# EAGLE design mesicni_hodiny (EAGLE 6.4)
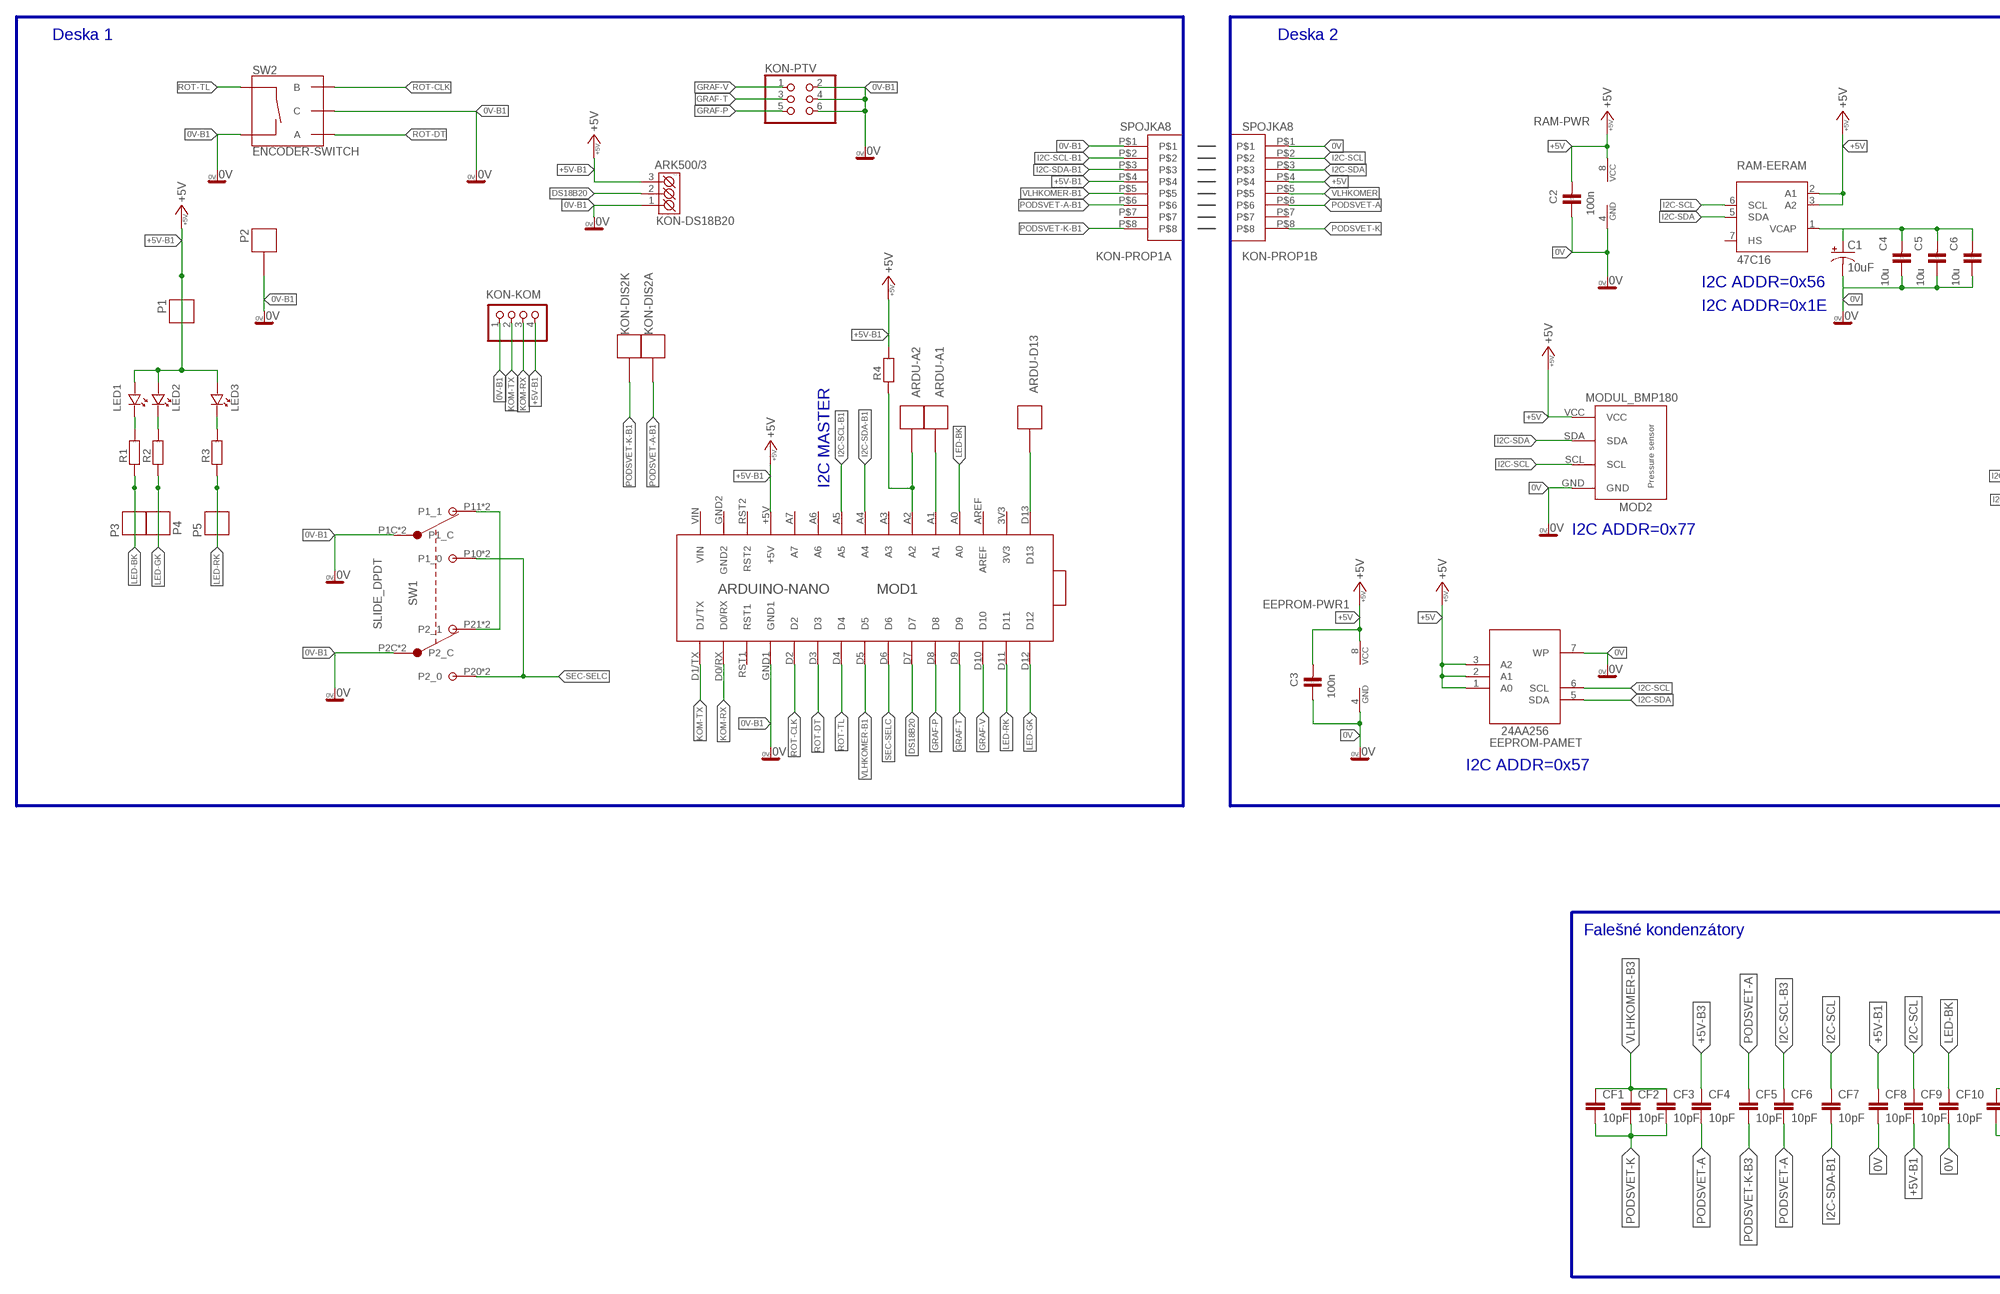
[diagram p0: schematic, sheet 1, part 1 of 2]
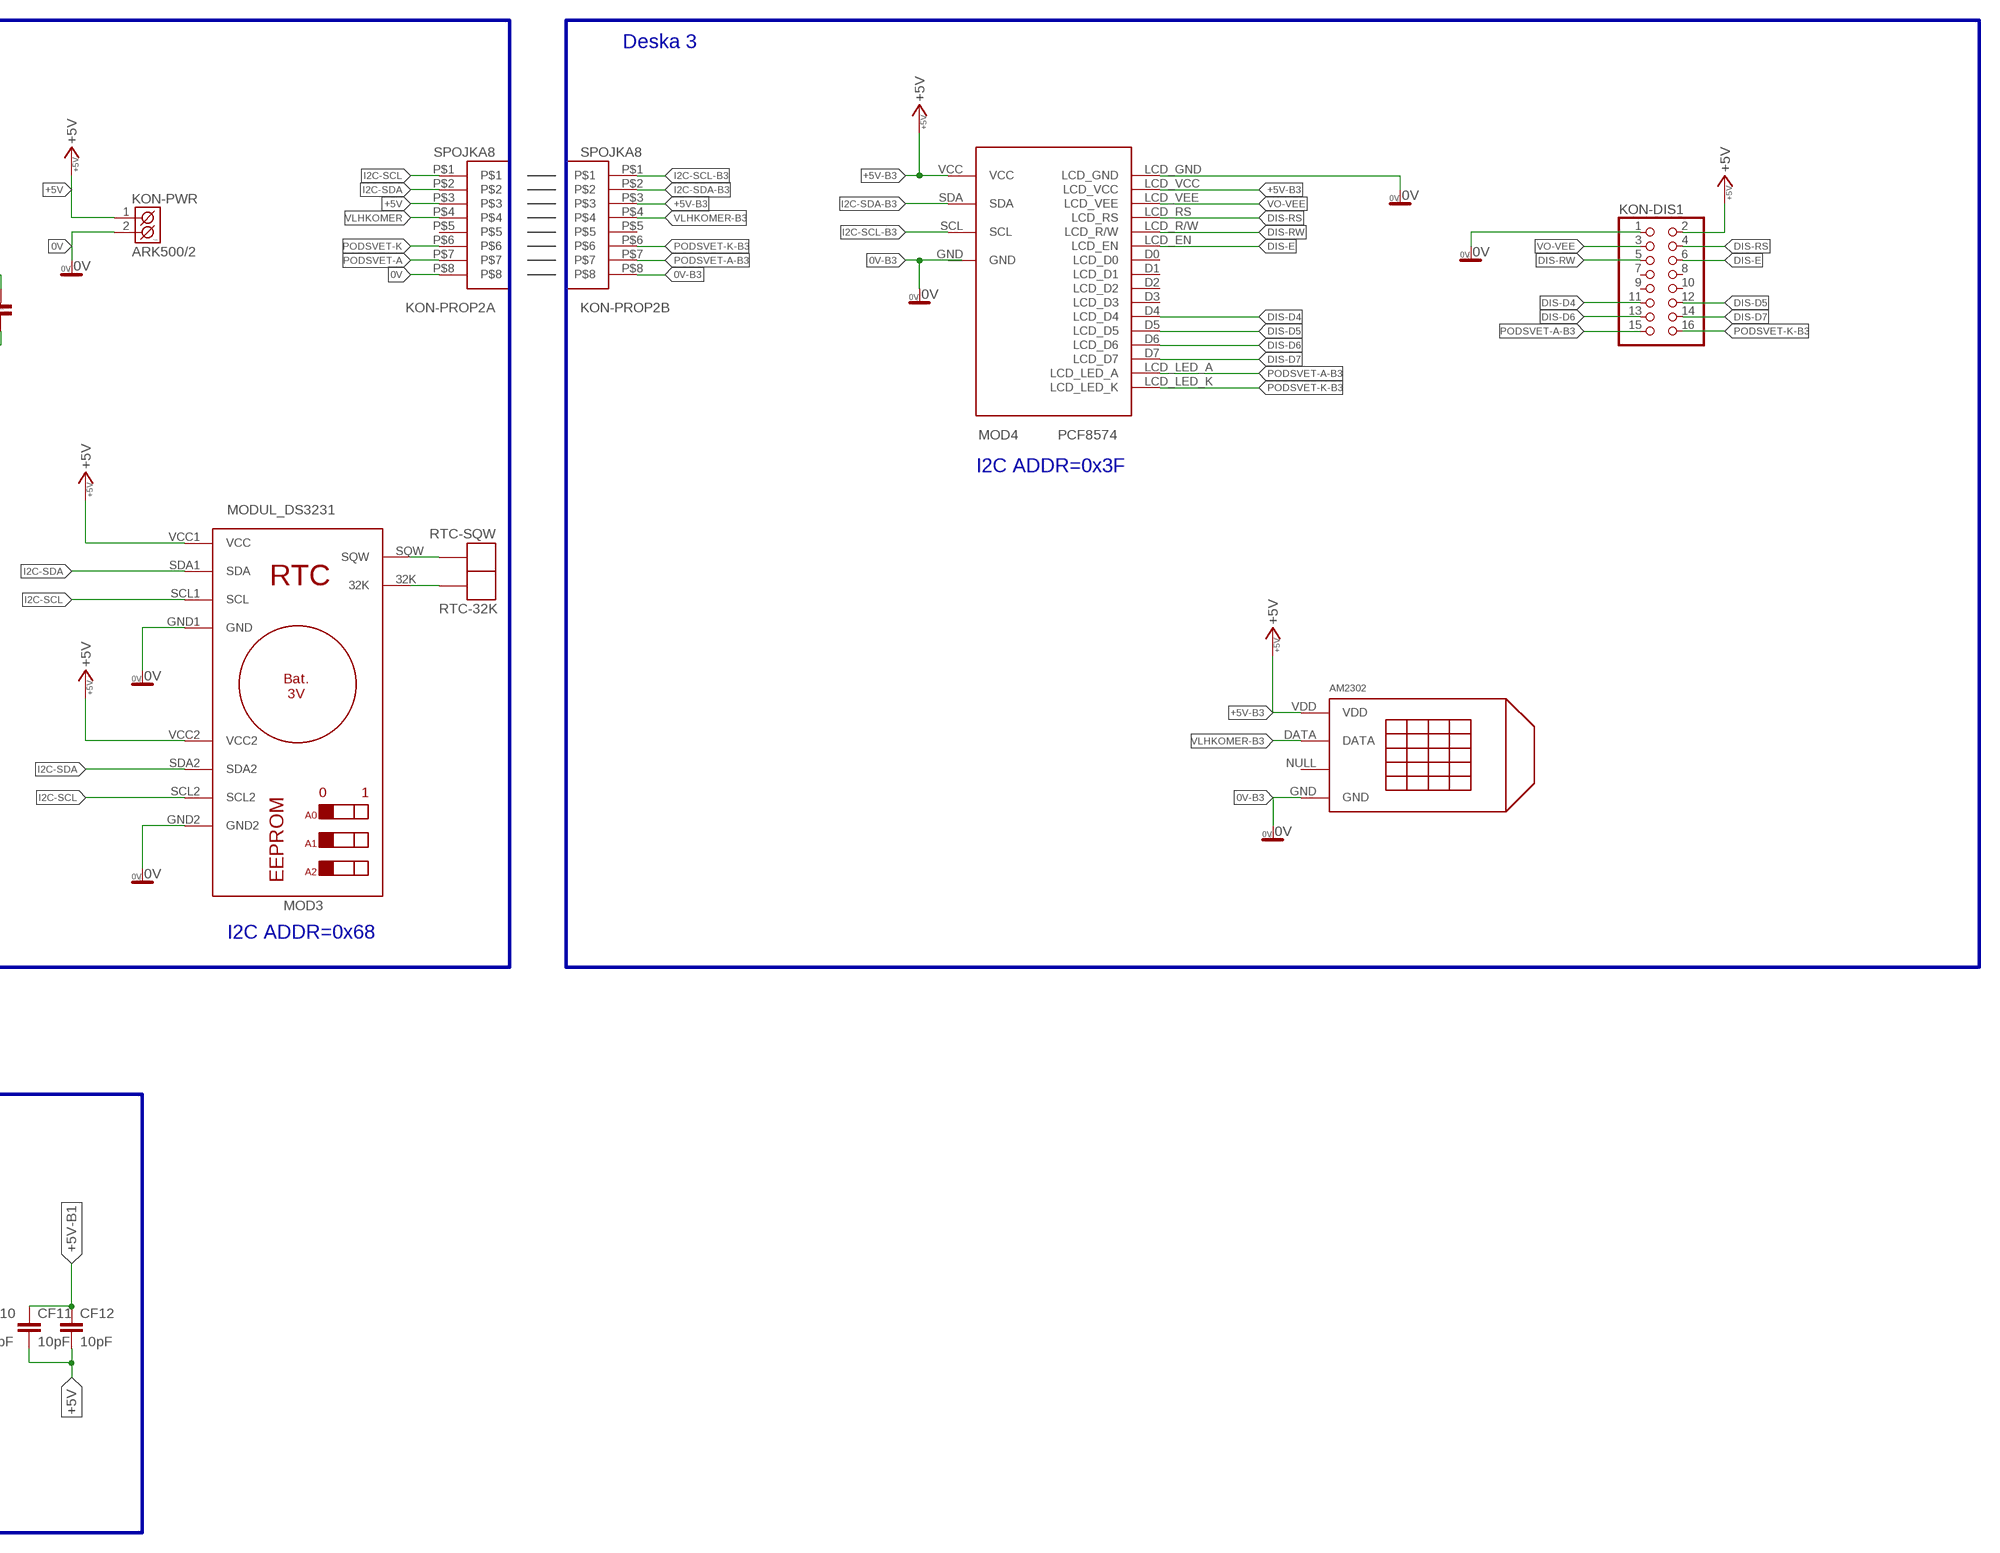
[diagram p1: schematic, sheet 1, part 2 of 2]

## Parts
AM2302  RHT03_DHT-22_AM2302RA  [RHT03_DHT-22/RA]
ARDU-A1  BIGPIN  [BIGPIN]
ARDU-A2  BIGPIN  [BIGPIN]
ARDU-D13  BIGPIN  [BIGPIN]
C1  10uF  10UF-POLAR-RADIAL-2.5MM-25V-20%  [CPOL-RADIAL-2.5MM-5MM]
C2  100n  C-KERAMIK_SMD_0805  [0805]
C3  100n  C-KERAMIK_SMD_0805  [0805]
C4  10u  C-KERAMIK_SMD_0805  [0805]
C5  10u  C-KERAMIK_SMD_0805  [0805]
C6  10u  C-KERAMIK_SMD_0805  [0805]
CF1  10pF  10PF-0603-50V-5%  [0603]
CF2  10pF  10PF-0603-50V-5%  [0603]
CF3  10pF  10PF-0603-50V-5%  [0603]
CF4  10pF  10PF-0603-50V-5%  [0603]
CF5  10pF  10PF-0603-50V-5%  [0603]
CF6  10pF  10PF-0603-50V-5%  [0603]
CF7  10pF  10PF-0603-50V-5%  [0603]
CF8  10pF  10PF-0603-50V-5%  [0603]
CF9  10pF  10PF-0603-50V-5%  [0603]
CF10  10pF  10PF-0603-50V-5%  [0603]
CF11  10pF  10PF-0603-50V-5%  [0603]
CF12  10pF  10PF-0603-50V-5%  [0603]
EEPROM  24AA256  EEPROMP  [DIL08]
KON-DIS1  PINHD-2X8  [2X08]
KON-DIS2A  BIGPIN  [BIGPIN]
KON-DIS2K  BIGPIN  [BIGPIN]
KON-DS18B20  ARK500/3  [ARK500/3]
KON-KOM  PINHD-1X4  [1X04]
KON-PROP1A  SPOJKA8  [SPOJKA8]
KON-PROP1B  SPOJKA8  [SPOJKA8]
KON-PROP2A  SPOJKA8  [SPOJKA8]
KON-PROP2B  SPOJKA8  [SPOJKA8]
KON-PTV  PINHD-2X3  [2X03]
KON-PWR  ARK500/2  [ARK500/2]
LED1  LED_3  [LED_3]
LED2  LED_3  [LED_3]
LED3  LED_3  [LED_3]
MOD1  ARDUINO-NANO  [PDIP-32]
MOD2  MODUL_BMP180  [MODUL_BMP180]
MOD3  MODUL_DS3231  [DS3231]
MOD4  PCF8574  I2C_DISPLAY_BACKPACK  [I2C_DISPLAY_BACKPACK]
P1  BIGPIN  [BIGPIN]
P2  BIGPIN  [BIGPIN]
P3  BIGPIN  [BIGPIN]
P4  BIGPIN  [BIGPIN]
P5  BIGPIN  [BIGPIN]
R1  R_SMD_0805  [0805]
R2  R_SMD_0805  [0805]
R3  R_SMD_0805  [0805]
R4  R_SMD_0805  [0805]
RAM  47C16  PCA8581CT  [SO08]
RTC-32K  BIGPIN  [BIGPIN]
RTC-SQW  BIGPIN  [BIGPIN]
SW1  SLIDE_DPDT  [SLIDE_DPDT]
SW2  ENCODER-SWITCH  [ROTARY_ENC_PLAIN]

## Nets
0V: C1.2(-) C2.1 C3.1 C4.1 C5.1 C6.1 CF8.2 CF10.2 EEPROM.4(-PWR1:GND) EEPROM.7(-PAMET:WP) KON-PROP1B.P$1 KON-PROP2A.P$8 KON-PWR.2(K2) MOD2.GND MOD3.GND1(GND) MOD3.GND2 RAM.4(-PWR:GND)
0V-B1: KON-DS18B20.1(K1) KON-KOM.1 KON-PROP1A.P$1 KON-PTV.2 KON-PTV.4 KON-PTV.6 MOD1.GND1 P2.P$1 SW1.P1C(P1_C) SW1.P1CSMD(P1_C) SW1.P2C(P2_C) SW1.P2CSMD(P2_C) SW2.C SW2.SW- ; supply symbol labelled 0V
0V-B3: AM2302.GND KON-DIS1.1 KON-PROP2B.P$8 MOD4.GND MOD4.LCD_GND ; supply symbol labelled 0V
+5V: C2.2 C3.2 CF11.2 CF12.2 EEPROM.1(-PAMET:A0) EEPROM.2(-PAMET:A1) EEPROM.3(-PAMET:A2) EEPROM.8(-PWR1:VCC) KON-PROP1B.P$4 KON-PROP2A.P$3 KON-PWR.1(K1) MOD2.VCC MOD3.VCC1(VCC) MOD3.VCC2 RAM.2(-EERAM:A1) RAM.3(-EERAM:A2) RAM.8(-PWR:VCC)
+5V-B1: CF8.1 CF9.2 CF11.1 CF12.1 KON-DS18B20.3(K3) KON-KOM.4 KON-PROP1A.P$4 LED1.A LED2.A LED3.A MOD1.+5V P1.P$1 R4.2 ; supply symbol labelled +5V
+5V-B3: AM2302.VDD CF4.1 KON-DIS1.2 KON-PROP2B.P$3 MOD4.LCD_VCC MOD4.VCC ; supply symbol labelled +5V
A1: ARDU-A1.P$1 MOD1.A1
DIS-D4: KON-DIS1.11 MOD4.D4(LCD_D4)
DIS-D5: KON-DIS1.12 MOD4.D5(LCD_D5)
DIS-D6: KON-DIS1.13 MOD4.D6(LCD_D6)
DIS-D7: KON-DIS1.14 MOD4.D7(LCD_D7)
DIS-E: KON-DIS1.6 MOD4.LCD_EN
DIS-RS: KON-DIS1.4 MOD4.LCD_RS
DIS-RW: KON-DIS1.5 MOD4.LCD_R/W
DS18B20: KON-DS18B20.2(K2) MOD1.D7
GRAF-P: KON-PTV.5 MOD1.D8
GRAF-T: KON-PTV.3 MOD1.D9
GRAF-V: KON-PTV.1 MOD1.D10
I2C-SCL: CF7.1 CF9.1 EEPROM.6(-PAMET:SCL) KON-PROP1B.P$2 KON-PROP2A.P$1 MOD2.SCL MOD3.SCL1(SCL) MOD3.SCL2 RAM.6(-EERAM:SCL)
I2C-SCL-B1: KON-PROP1A.P$2 MOD1.A5
I2C-SCL-B3: CF6.1 KON-PROP2B.P$1 MOD4.SCL
I2C-SDA: EEPROM.5(-PAMET:SDA) KON-PROP1B.P$3 KON-PROP2A.P$2 MOD2.SDA MOD3.SDA1(SDA) MOD3.SDA2 RAM.5(-EERAM:SDA)
I2C-SDA-B1: CF7.2 KON-PROP1A.P$3 MOD1.A4
I2C-SDA-B3: KON-PROP2B.P$2 MOD4.SDA
KOM-RX: KON-KOM.3 MOD1.D0/RX
KOM-TX: KON-KOM.2 MOD1.D1/TX
LED-BK: CF10.1 MOD1.A0 P3.P$1 R1.1
LED-GK: MOD1.D12 P4.P$1 R2.1
LED-RK: MOD1.D11 P5.P$1 R3.1
N$1: LED1.K R1.2
N$2: LED2.K R2.2
N$3: LED3.K R3.2
N$5: MOD3.SQW RTC-SQW.P$1
N$7: MOD3.32K RTC-32K.P$1
N$8: ARDU-D13.P$1 MOD1.D13
N$9: ARDU-A2.P$1 MOD1.A2 R4.1
N$17: C1.1(+) C4.2 C5.2 C6.2 RAM.1(-EERAM:VCAP)
NIC-1: SW1.P11(P1_1) SW1.P11SMD(P1_1) SW1.P21(P2_1) SW1.P21SMD(P2_1)
PODSVET-A: CF4.2 CF5.1 CF6.2 KON-PROP1B.P$6 KON-PROP2A.P$7
PODSVET-A-B1: KON-DIS2A.P$1 KON-PROP1A.P$6
PODSVET-A-B3: KON-DIS1.15 KON-PROP2B.P$7 MOD4.LCD_LED_A
PODSVET-K: CF1.2 CF2.2 CF3.2 KON-PROP1B.P$8 KON-PROP2A.P$6
PODSVET-K-B1: KON-DIS2K.P$1 KON-PROP1A.P$8
PODSVET-K-B3: CF5.2 KON-DIS1.16 KON-PROP2B.P$6 MOD4.LCD_LED_K
ROT-CLK: MOD1.D2 SW2.B
ROT-DT: MOD1.D3 SW2.A
ROT-TL: MOD1.D4 SW2.SW+
SEC-SELC: MOD1.D6 SW1.P10(P1_0) SW1.P10SMD(P1_0) SW1.P20(P2_0) SW1.P20SMD(P2_0)
VLHKOMER: KON-PROP1B.P$5 KON-PROP2A.P$4
VLHKOMER-B1: KON-PROP1A.P$5 MOD1.D5
VLHKOMER-B3: AM2302.DATA CF1.1 CF2.1 CF3.1 KON-PROP2B.P$4
VO-VEE: KON-DIS1.3 MOD4.LCD_VEE
Unconnected: AM2302.NULL KON-DIS1.7 KON-DIS1.8 KON-DIS1.9 KON-DIS1.10 KON-PROP1A.P$7 KON-PROP1B.P$7 KON-PROP2A.P$5 KON-PROP2B.P$5 MOD1.3V3 MOD1.A3 MOD1.A6 MOD1.A7 MOD1.AREF MOD1.GND2 MOD1.RST1 MOD1.RST2 MOD1.VIN MOD4.D0(LCD_D0) MOD4.D1(LCD_D1) MOD4.D2(LCD_D2) MOD4.D3(LCD_D3) RAM.7(-EERAM:HS)

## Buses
B$1
B$2
B$3
B$4

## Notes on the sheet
- Deska 1 | Deska 2 | Deska 3
- I2C ADDR=0x56
- I2C ADDR=0x1E
- I2C ADDR=0x3F
- I2C MASTER
- I2C ADDR=0x77
- I2C ADDR=0x57
- I2C ADDR=0x68
- Falešné kondenzátory

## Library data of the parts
AM2302 = RHT03_DHT-22_AM2302:RHT03_DHT-22_AM2302: RHT03 / DHT-22 / AM2302 Packages and symbol for the RHT03 / DHT-22 relative humidity and temperature sensor. Note: The AM2302 is a wired version of the DHT-22 which typically requires less clearance and is thus provided as a separate package.; PROD_ID: SEN-10167
ARDU-A1 ARDU-A2 ARDU-D13 KON-DIS2A KON-DIS2K P1-P5 RTC-32K RTC-SQW = bigpin:BIGPIN: Jeden ovalny pin
C1 = SparkFun-Capacitors:10UF-POLAR: 10.0µF polarized capacitors; PROD_ID: CAP-08440
C2-C6 = #PaJa_30:C-KERAMIK: Kondenzator - keramicky
CF1-CF12 = SparkFun-Capacitors:10PF: 10pF ceramic capacitors; PROD_ID: CAP-11812
EEPROM = eeprom:EEPROM: EEPROM
KON-DIS1 = pinhead:PINHD-2X8: PIN HEADER
KON-DS18B20 = #PaJa_konektory:ARK500/3: Svorkovnice - roztec 5mm - trojita
KON-KOM = pinhead:PINHD-1X4: PIN HEADER
KON-PROP1A KON-PROP1B KON-PROP2A KON-PROP2B = spopjka8:SPOJKA8
KON-PTV = pinhead:PINHD-2X3: PIN HEADER
KON-PWR = #PaJa_konektory:ARK500/2: Svorkovnice - roztec 5mm - dvojita
LED1-LED3 = #PaJa_30:LED: LED - jednobarevna
MOD1 = jet-lib:ARDUINO-NANO: Arduino NANO - V3
MOD2 = modul_bmp180:MODUL_BMP180
MOD3 = modul_DS3231:MODUL_DS3231: Modul DS3231 s externi pameti
MOD4 = i2c_display_backpack:I2C_DISPLAY_BACKPACK
R1-R4 = #PaJa_30:R: Rezistor
RAM = i2c:PCA8581: 2048 x 8-Bit EERAM with I²C Bus Interface
SW1 = slide_DPDT:SLIDE_DPDT
SW2 = SparkFun-Switches:ENCODER-SWITCH: Rotary Encoder w/ Select Switch Encoders rotate similarly to potentiometers, but they’re different from potentiometers in that an encoder has full rotation without limits. They output gray code so that you can tell how much and in which direction the encoder has been turned. This encoder includes a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; SF_SKU: COM-09117

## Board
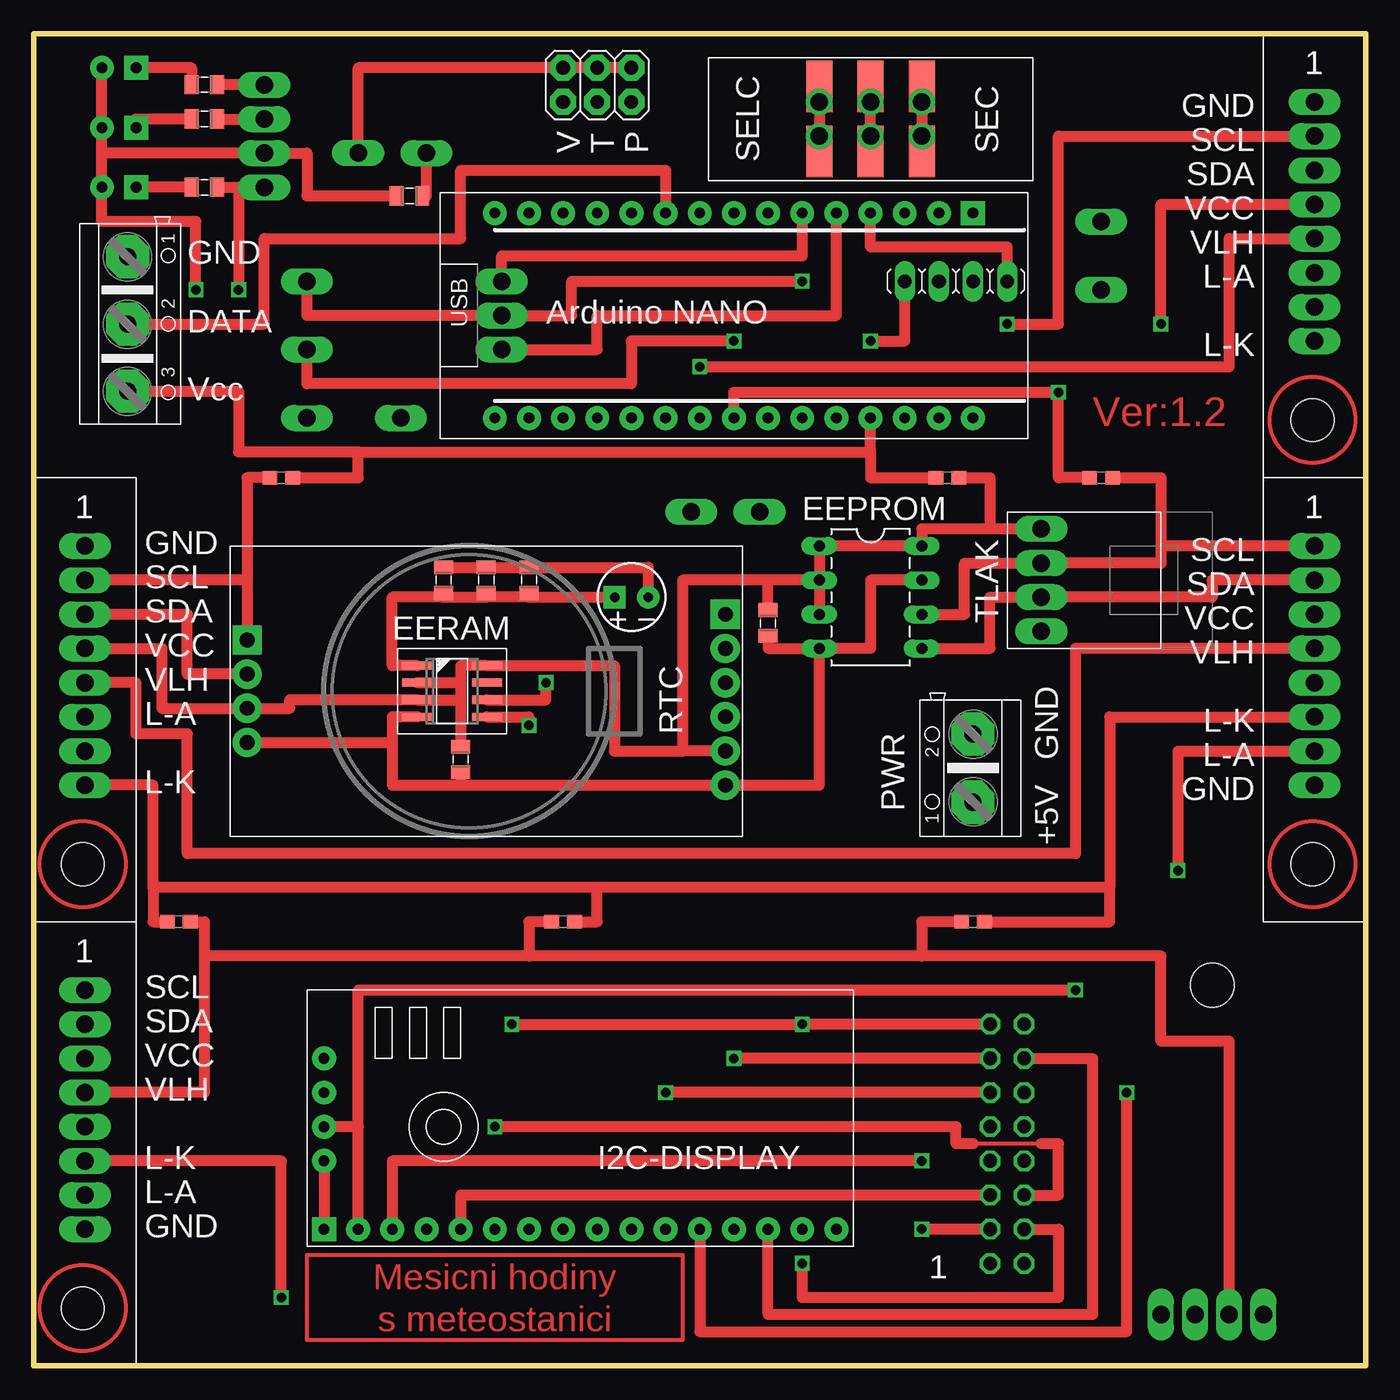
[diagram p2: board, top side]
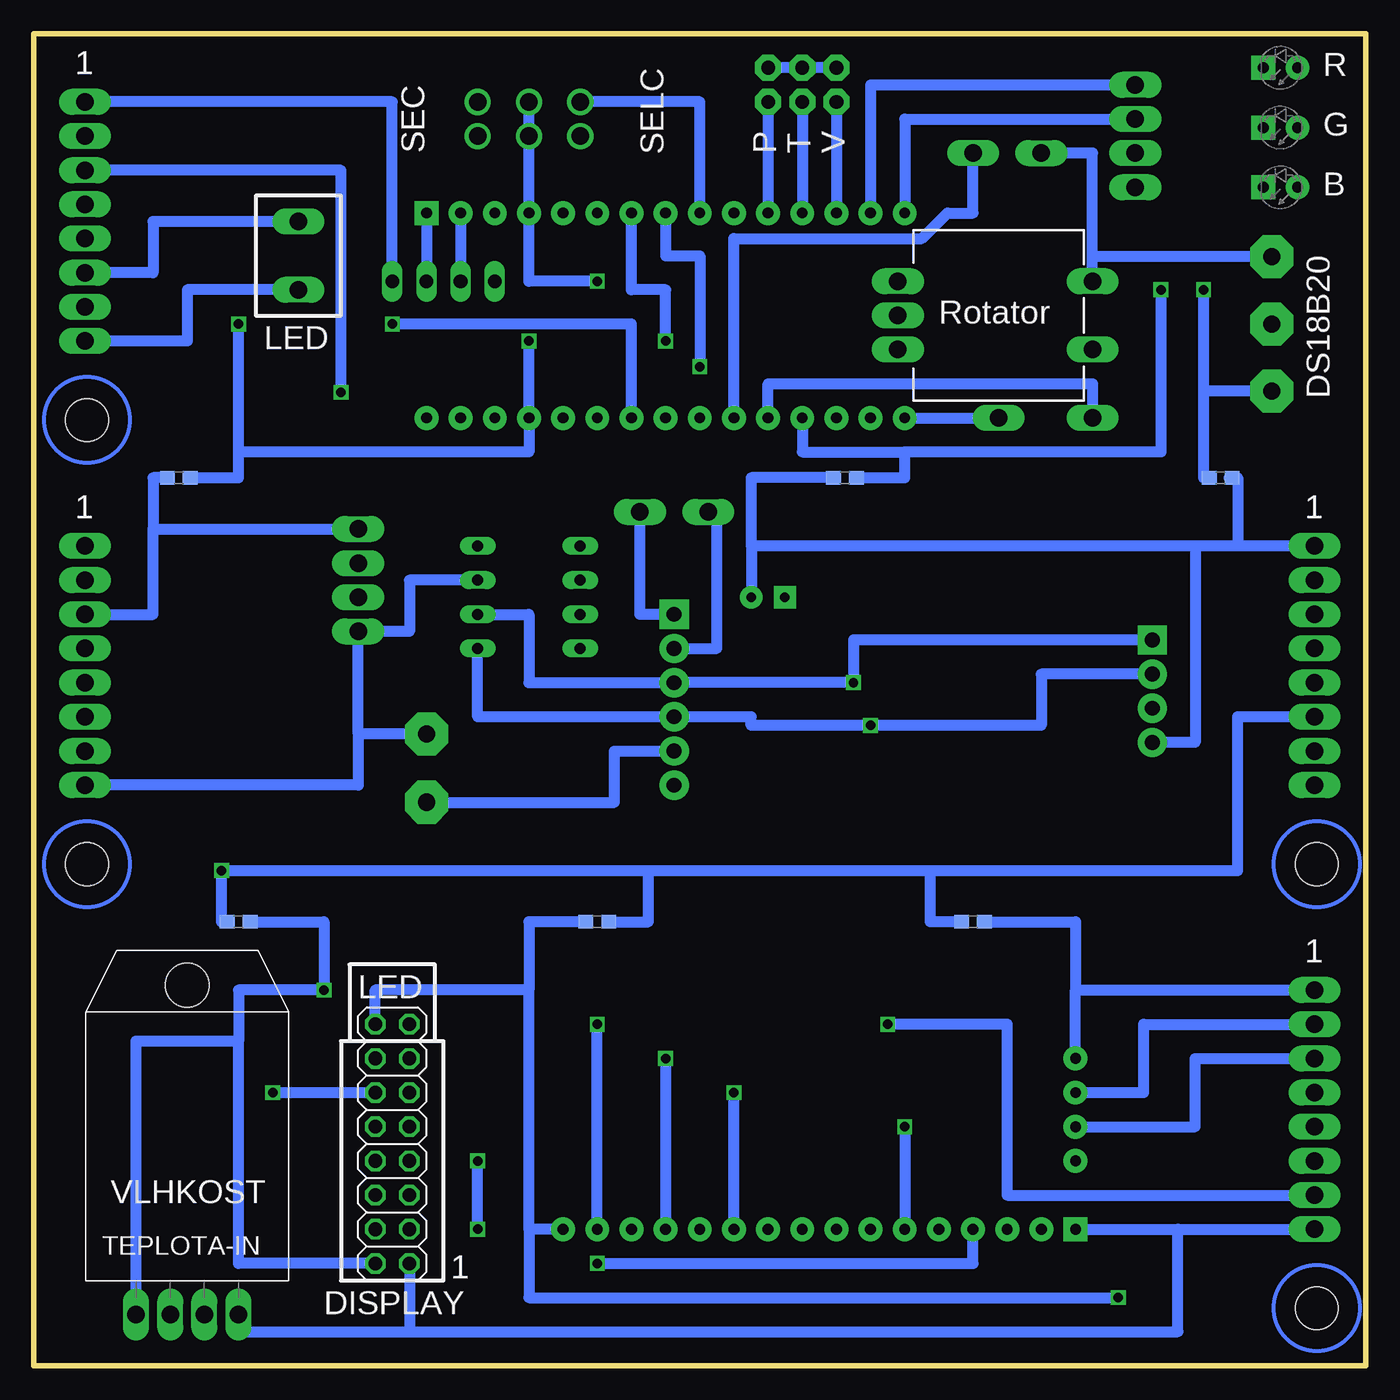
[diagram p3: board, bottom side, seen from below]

Size 99.06 x 99.06 mm. Coordinates in mm from the lower left corner, seen from the top.
Outline: 0,99.06 99.06,99.06 99.06,0 0,0 0,99.06
Copper layers (1*16): Top 0.035mm / dielectric 1.5mm / Bottom 0.035mm
Design rules "default *": minimum track width 10mil, minimum drill 24mil, track to track 8mil, track to pad 8mil, pad to pad 8mil, via to via 8mil, smd to smd 8mil, copper to edge 40mil, drill to drill 8mil, minimum pad ring 10mil, minimum via ring 8mil, stop-mask expansion 4mil, vias tented up to drill 0mil, thermal gap 10mil

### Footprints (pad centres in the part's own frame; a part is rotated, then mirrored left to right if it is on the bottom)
RHT03_DHT-22/RA = drill 1.3 pad 1.778 long: DATA -1.27,0; GND 3.81,0; NULL 1.27,0; VDD -3.81,0 | hole 3.25: 0,24.5
BIGPIN = drill 1.3 long: P$1 0,0
CPOL-RADIAL-2.5MM-5MM = drill 0.7 pad 1.651 square: 1 1.25,0 | drill 0.7 pad 1.651: 2 -1.25,0
0805 = smd 1.016 x 1.422: 1 -0.953,0; 2 0.953,0
0603 = smd 1.1 x 1: 1 -0.85,0; 2 0.85,0
DIL08 = drill 0.813 long: 1 -3.81,-3.81; 2 -1.27,-3.81; 3 1.27,-3.81; 4 3.81,-3.81; 5 3.81,3.81; 6 1.27,3.81; 7 -1.27,3.81; 8 -3.81,3.81
2X08 = drill 1.016 octagon: 1 -8.89,-1.27; 2 -8.89,1.27; 3 -6.35,-1.27; 4 -6.35,1.27; 5 -3.81,-1.27; 6 -3.81,1.27; 7 -1.27,-1.27; 8 -1.27,1.27; 9 1.27,-1.27; 10 1.27,1.27; 11 3.81,-1.27; 12 3.81,1.27; 13 6.35,-1.27; 14 6.35,1.27; 15 8.89,-1.27; 16 8.89,1.27
ARK500/3 = drill 1.27 pad 3.2 octagon: 1 -5,0; 2 0,0; 3 5,0
1X04 = drill 1.016 long: 1 -3.81,0; 2 -1.27,0; 3 1.27,0; 4 3.81,0
SPOJKA8 = drill 1.3 pad 1.778 long: P$1 0,8.89; P$2 0,6.35; P$3 0,3.81; P$4 0,1.27; P$5 0,-1.27; P$6 0,-3.81; P$7 0,-6.35; P$8 0,-8.89 | hole 3.2: -0.159,-14.764
2X03 = drill 1.016 pad 1.93 octagon: 1 -2.54,-1.27; 2 -2.54,1.27; 3 0,-1.27; 4 0,1.27; 5 2.54,-1.27; 6 2.54,1.27
ARK500/2 = drill 1.27 pad 3.2 octagon: 1 -2.54,0; 2 2.54,0
LED_3 = drill 0.813 pad 1.778: A -1.27,0 | drill 0.813 pad 1.778 square: K 1.27,0
PDIP-32 = drill 0.8 pad 1.778: 3V3 15.24,-35.56; +5V 15.24,-10.16; A0 15.24,-30.48; A1 15.24,-27.94; A2 15.24,-25.4; A3 15.24,-22.86; A4 15.24,-20.32; A5 15.24,-17.78; A6 15.24,-15.24; A7 15.24,-12.7; AREF 15.24,-33.02; D0/RX 0,-5.08; D2 0,-12.7; D3 0,-15.24; D4 0,-17.78; D5 0,-20.32; D6 0,-22.86; D7 0,-25.4; D8 0,-27.94; D9 0,-30.48; D10 0,-33.02; D11 0,-35.56; D12 0,-38.1; D13 15.24,-38.1; GND1 0,-10.16; GND2 15.24,-5.08; RST1 0,-7.62; RST2 15.24,-7.62; VIN 15.24,-2.54 | drill 0.8 pad 1.778 square: D1/TX 0,-2.54
MODUL_BMP180 = drill 1.3 pad 1.778 long: GND -3.81,3.81; SCL 1.27,3.81; SDA -1.27,3.81; VCC 3.81,3.81
DS3231 = drill 1.1 pad 2.184 square: 32K 36.83,16.51; SCL1 1.27,14.605 | drill 1.1 pad 2.184: GND1 1.27,6.985; GND2 36.83,3.81; SCL2 36.83,11.43; SDA1 1.27,12.065; SDA2 36.83,8.89; SQW 36.83,13.97; VCC1 1.27,9.525; VCC2 36.83,6.35
I2C_DISPLAY_BACKPACK = drill 0.8 pad 1.778: D0 5.08,7.62; D1 2.54,7.62; D2 0,7.62; D3 -2.54,7.62; D4 -5.08,7.62; D5 -7.62,7.62; D6 -10.16,7.62; D7 -12.7,7.62; GND 20.32,2.54; LCD_EN 7.62,7.62; LCD_LED_A -15.24,7.62; LCD_LED_K -17.78,7.62; LCD_R/W 10.16,7.62; LCD_RS 12.7,7.62; LCD_VCC 17.78,7.62; LCD_VEE 15.24,7.62; SCL 20.32,-5.08; SDA 20.32,-2.54; VCC 20.32,0 | drill 0.8 pad 1.778 square: LCD_GND 20.32,7.62
SO08 = smd 0.6 x 2.2: 1 -1.905,-2.6; 2 -0.635,-2.6; 3 0.635,-2.6; 4 1.905,-2.6; 5 1.905,2.6; 6 0.635,2.6; 7 -0.635,2.6; 8 -1.905,2.6
SLIDE_DPDT = drill 1.3: P1C -1.27,0; P2C 1.27,0; P10 -1.27,3.81; P11 -1.27,-3.81; P20 1.27,3.81; P21 1.27,-3.81 | smd 3.81 x 1.93: P1CSMD -2.413,0; P2CSMD 2.413,0; P10SMD -2.413,3.81; P11SMD -2.413,-3.81; P20SMD 2.413,3.81; P21SMD 2.413,-3.81
ROTARY_ENC_PLAIN = drill 1.3 pad 1.778 long: A 7.493,-2.54; B 7.493,2.54; C 7.493,0; SW+ -6.985,2.54; SW- -6.985,-2.54

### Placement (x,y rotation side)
AM2302  87.63,3.81 0 bottom
ARDU-A1  20.32,70.48 0 top
ARDU-A2  29.21,90.17 0 top
ARDU-D13  27.3,70.48 0 top
C1  44.45,57.15 180 top
C2  31.75,45.09 90 top
C3  54.61,55.24 90 top
C4  36.83,58.42 270 top
C5  33.66,58.42 270 top
C6  30.48,58.42 270 top
CF1  10.79,33.02 180 top
CF2  39.37,33.02 0 top
CF3  69.85,33.02 0 top
CF4  83.82,33.02 180 bottom
CF5  57.15,33.02 180 bottom
CF6  29.21,33.02 180 bottom
CF7  79.38,66.04 180 top
CF8  10.79,66.04 0 bottom
CF9  18.41,66.04 0 top
CF10  38.73,66.04 180 bottom
CF11  67.94,66.04 0 top
CF12  88.27,66.04 180 bottom
EEPROM  62.23,57.15 270 top
KON-DIS1  72.39,16.51 90 bottom
KON-DIS2A  79.38,85.09 0 top
KON-DIS2K  79.38,80.01 0 top
KON-DS18B20  6.99,77.47 270 top
KON-KOM  68.58,80.64 180 top
KON-PROP1A  95.25,85.09 0 top
KON-PROP1B  3.81,52.07 0 top
KON-PROP2A  95.25,52.07 0 top
KON-PROP2B  3.81,19.05 0 top
KON-PTV  41.91,95.25 0 top
KON-PWR  69.85,44.45 90 top
LED1  6.35,87.63 180 bottom
LED2  6.35,92.08 180 bottom
LED3  6.35,96.52 180 bottom
MOD1  72.39,85.72 270 top
MOD2  78.74,58.42 90 top
MOD3  14.61,39.37 0 top
MOD4  41.91,17.78 180 top
P1  17.14,90.17 0 top
P2  24.13,90.17 180 top
P3  17.14,87.63 0 top
P4  17.14,92.71 0 top
P5  17.14,95.25 0 top
R1  12.7,87.63 180 top
R2  12.7,92.71 180 top
R3  12.7,95.25 180 top
R4  27.94,87 180 top
RAM  31.11,50.16 270 top
RTC-32K  53.98,63.5 180 top
RTC-SQW  48.9,63.5 180 top
SW1  62.23,92.71 90 top
SW2  27.3,78.11 180 bottom

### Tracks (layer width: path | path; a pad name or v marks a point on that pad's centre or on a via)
0V
  Top 0.813: EEPROM.7 62.23,58.42 62.23,53.34 EEPROM.4 | EEPROM.4 58.42,43.18 MOD3.GND2 31.75,43.18 | RAM.4 26.67,48.26 26.67,46.35 | 26.67,46.35 26.67,43.18 31.75,43.18 | MOD3.GND1 26.67,46.35 | C2.1 31.75,43.18 | C3.1 54.61,53.34 EEPROM.4 | C6.1 C5.1 C4.1 45.7,59.37 C1.2
  Bottom 0.813: 74.93,46.99 MOD2.GND 71.12,54.61 71.12,58.42 EEPROM.7 | 12.7,60.96 12.7,46.35 MOD3.GND1 | KON-PROP2A.P$8 74.93,43.18 74.93,46.99 | KON-PROP1B.P$1 9.53,60.96 | 10.16,66.04 CF8.2 9.53,66.04 9.53,60.96 | 9.53,60.96 12.7,60.96 | CF10.2 45.7,66.04 45.7,60.96 | KON-PWR.2 74.93,46.99 | 12.7,60.96 45.7,60.96 | 45.7,60.96 C1.2
0V-B1  (via drill 0.7)
  Top 0.813: v57.15,80.64 40.01,80.64 40.01,78.11 SW2.C 20.32,78.11 SW2.SW- | P2.P$1 24.13,96.52 KON-PTV.6 | SW1.P1CSMD SW1.P1C SW1.P2C SW1.P2CSMD | KON-KOM.1 72.39,83.19 62.23,83.19 MOD1.GND1
  Bottom 0.813: v57.15,80.64 62.23,80.64 MOD1.GND1 SW1.P2C | KON-KOM.1 72.39,93.98 KON-PROP1A.P$1 | KON-PTV.2 KON-PTV.4 KON-PTV.6 | 20.32,82.47 20.32,90.17 P2.P$1 | KON-DS18B20.1 20.32,82.47 | SW2.SW- 20.32,82.47
0V-B3
  Top 0.813: MOD4.GND MOD4.LCD_GND
  Bottom 0.813: AM2302.GND 83.82,2.54 71.12,2.54 | 71.12,2.54 13.97,2.54 13.97,10.16 | MOD4.LCD_GND 13.97,10.16 | 13.97,10.16 KON-PROP2B.P$8 | KON-DIS1.1 71.12,2.54
+5V
  Top 0.813: MOD2.VCC 71.12,62.23 | 71.12,62.23 66.04,62.23 EEPROM.8 EEPROM.1 EEPROM.2 | EEPROM.2 EEPROM.3 | EEPROM.2 54.61,58.42 | 54.61,58.42 48.26,58.42 48.26,45.72 | 48.26,45.72 43.18,45.72 43.18,52.07 RAM.8 31.75,52.07 31.75,50.8 | MOD3.VCC2 48.26,45.72 | KON-PROP1B.P$4 9.53,53.34 9.53,48.9 MOD3.VCC1 19.05,48.9 19.05,49.53 RAM.3 31.75,49.53 | 31.75,50.8 31.75,49.53 | 31.75,49.53 C2.2 | C3.2 54.61,58.42 | RAM.2 31.75,50.8 | CF11.2 71.12,66.04 71.12,62.23
  Bottom 0.813: KON-PROP2A.P$3 90.17,55.88 90.17,62.23 | 90.17,62.23 MOD2.VCC | CF12.2 90.17,66.04 90.17,62.23 | KON-PWR.1 55.88,41.91 55.88,45.72 MOD3.VCC2
+5V-B1  (via drill 0.7)
  Top 0.813: v83.82,77.47 83.82,86.36 KON-PROP1A.P$4 | KON-DS18B20.3 15.24,72.47 15.24,67.94 24.13,67.94 | 24.13,67.94 62.23,67.94 | 62.23,67.94 MOD1.+5V | v12.06,80.01 12.06,85.09 5.08,85.09 LED1.A 5.08,90.17 | CF9.2 24.13,66.04 24.13,67.94 | 62.23,67.94 62.23,66.04 CF11.1 | v62.23,76.2 64.77,76.2 KON-KOM.4 | 5.08,90.17 LED2.A LED3.A | 5.08,90.17 P1.P$1 20.32,90.17 20.32,87 R4.2
  Bottom 0.813: 83.82,67.94 62.23,67.94 MOD1.+5V v62.23,76.2 | 83.82,67.94 v83.82,77.47 | KON-DS18B20.3 12.06,72.47 | 12.06,72.47 v12.06,80.01 | CF8.1 12.06,66.04 12.06,72.47 | CF12.1 83.82,66.04 83.82,67.94
+5V-B3  (via drill 0.7)
  Top 0.813: 24.13,17.78 MOD4.VCC | 24.13,17.78 24.13,27.94 v77.47,27.94 | MOD4.LCD_VCC 24.13,17.78
  Bottom 0.813: MOD4.VCC 12.7,17.78 12.7,22.86 KON-PROP2B.P$3 | 83.82,24.13 83.82,27.94 v77.47,27.94 77.47,33.02 CF4.1 | 83.82,24.13 91.44,24.13 AM2302.VDD | 83.82,24.13 83.82,7.62 KON-DIS1.2
A1
  Bottom 0.813: MOD1.A1 44.45,73.03 20.32,73.03 ARDU-A1.P$1
DIS-D4  (via drill 0.7)
  Top 0.813: KON-DIS1.11 v46.99,20.32
  Bottom 0.813: MOD4.D4 v46.99,20.32
DIS-D5  (via drill 0.7)
  Top 0.813: MOD4.D5 49.53,2.54 81.28,2.54 v81.28,20.32
  Bottom 0.813: v81.28,20.32 KON-DIS1.12
DIS-D6  (via drill 0.7)
  Top 0.813: KON-DIS1.13 v52.07,22.86
  Bottom 0.813: v52.07,22.86 MOD4.D6
DIS-D7
  Top 0.813: KON-DIS1.14 78.74,22.86 78.74,3.81 54.61,3.81 MOD4.D7
DIS-E  (via drill 0.7)
  Top 0.305: 74.93,16.51 69.85,16.51
  Top 0.813: KON-DIS1.6 76.2,12.7 76.2,16.51 74.93,16.51 | 69.85,16.51 68.58,16.51 68.58,17.78 v34.29,17.78
  Bottom 0.813: v34.29,17.78 MOD4.LCD_EN
DIS-RS  (via drill 0.7)
  Top 0.813: KON-DIS1.4 76.2,10.16 76.2,5.08 57.15,5.08 v57.15,7.62
  Bottom 0.813: v57.15,7.62 29.21,7.62 MOD4.LCD_RS
DIS-RW
  Top 0.813: KON-DIS1.5 31.75,12.7 MOD4.LCD_R/W
DS18B20
  Top 0.813: KON-DS18B20.2 17.14,77.47 17.14,83.82 31.75,83.82 31.75,88.9 46.99,88.9 MOD1.D7
GRAF-P
  Bottom 0.813: KON-PTV.5 MOD1.D8
GRAF-T
  Bottom 0.813: KON-PTV.3 MOD1.D9
GRAF-V
  Bottom 0.813: KON-PTV.1 MOD1.D10
I2C-SCL  (via drill 0.7)
  Top 0.813: KON-PROP2A.P$1 83.82,60.96 | 83.82,60.96 83.82,59.69 MOD2.SCL 69.22,59.69 69.22,55.88 EEPROM.6 | v38.1,50.8 38.1,49.53 RAM.6 | 15.88,58.42 MOD3.SCL1 | 15.88,58.42 KON-PROP1B.P$2 | CF9.1 15.88,66.04 15.88,58.42 | CF7.1 83.82,66.04 83.82,60.96
  Bottom 0.813: EEPROM.6 62.23,55.88 62.23,50.8 MOD3.SCL2 v38.1,50.8 38.1,53.98 MOD3.SCL1
I2C-SCL-B1  (via drill 0.7)
  Top 0.813: v72.39,77.47 76.2,77.47 76.2,91.44 KON-PROP1A.P$2
  Bottom 0.813: MOD1.A5 54.61,77.47 v72.39,77.47
I2C-SCL-B3
  Bottom 0.813: MOD4.SCL 21.59,27.94 | 21.59,27.94 KON-PROP2B.P$1 | CF6.1 21.59,33.02 21.59,27.94
I2C-SDA  (via drill 0.7)
  Top 0.813: KON-PROP2A.P$2 87.63,58.42 87.63,57.15 MOD2.SDA 71.12,57.15 71.12,53.34 EEPROM.5 | MOD3.SDA1 11.43,51.44 11.43,55.88 KON-PROP1B.P$3 | v36.83,47.62 36.83,48.26 RAM.5
  Bottom 0.813: MOD3.SDA1 24.13,51.44 24.13,47.62 v36.83,47.62 45.72,47.62 45.72,48.26 MOD3.SDA2 66.04,48.26 EEPROM.5
I2C-SDA-B1  (via drill 0.7)
  Top 0.813: MOD1.A4 52.07,72.39 v76.2,72.39 76.2,66.04 CF7.2
  Bottom 0.813: v76.2,72.39 76.2,88.9 KON-PROP1A.P$3
I2C-SDA-B3
  Bottom 0.813: MOD4.SDA 16.51,20.32 16.51,25.4 KON-PROP2B.P$2
KOM-RX
  Bottom 0.813: MOD1.D0/RX KON-KOM.3
KOM-TX
  Bottom 0.813: MOD1.D1/TX KON-KOM.2
LED-BK  (via drill 0.7)
  Top 0.813: R1.1 P3.P$1 15.24,87.63 v15.24,80.01
  Bottom 0.813: v15.24,80.01 15.24,67.94 34.29,67.94 | CF10.1 34.29,66.04 34.29,67.94 | MOD1.A0 41.91,67.94 34.29,67.94
LED-GK
  Top 0.813: R2.1 P4.P$1
  Bottom 0.813: MOD1.D12 34.29,92.71 P4.P$1
LED-RK
  Top 0.813: P5.P$1 R3.1
  Bottom 0.813: MOD1.D11 36.83,95.25 P5.P$1
N$1
  Top 0.813: R1.2 LED1.K
N$2
  Top 0.813: R2.2 7.62,92.71 LED2.K
N$3
  Top 0.813: R3.2 11.75,96.52 LED3.K
N$4
  Top 0.305: 20.32,8.26 48.26,8.26 48.26,1.91 20.32,1.91 20.32,8.26
N$5
  Bottom 0.813: MOD3.SQW 48.26,53.34 48.26,63.5 RTC-SQW.P$1
N$7
  Bottom 0.813: MOD3.32K 53.98,55.88 RTC-32K.P$1
N$8
  Bottom 0.813: MOD1.D13 ARDU-D13.P$1
N$9
  Top 0.813: R4.1 29.21,87 ARDU-A2.P$1
  Bottom 0.813: MOD1.A2 46.99,83.82 33.02,83.82 31.11,85.72 29.21,85.72 ARDU-A2.P$1
N$17
  Top 0.813: 36.83,57.15 C1.1 | RAM.1 26.67,52.07 26.67,57.15 30.48,57.15 | C4.2 36.83,57.15 | 36.83,57.15 33.66,57.15 | C6.2 30.48,57.15 | 30.48,57.15 33.66,57.15 | 33.66,57.15 C5.2
NIC-1
  Top 0.813: SW1.P11SMD SW1.P11 SW1.P21 SW1.P21SMD
PODSVET-A  (via drill 0.7)
  Top 0.813: v85.09,36.83 85.09,45.72 KON-PROP2A.P$7
  Bottom 0.813: 53.34,36.83 v85.09,36.83 85.09,33.02 CF4.2 | 53.34,36.83 32.38,36.83 | 32.38,36.83 9.53,36.83 9.53,48.26 KON-PROP1B.P$6 | CF5.1 53.34,33.02 53.34,36.83 | CF6.2 32.38,33.02 32.38,36.83
PODSVET-A-B1
  Bottom 0.813: KON-DIS2A.P$1 90.17,85.09 90.17,81.28 KON-PROP1A.P$6
PODSVET-A-B3  (via drill 0.7)
  Top 0.813: v35.56,25.4 v57.15,25.4 KON-DIS1.15
  Bottom 0.813: v35.56,25.4 26.67,25.4 26.67,12.7 KON-PROP2B.P$7 | MOD4.LCD_LED_A v57.15,25.4
PODSVET-K
  Top 0.813: 80.01,35.56 80.01,48.26 KON-PROP2A.P$6 | 80.01,35.56 41.91,35.56 | 41.91,35.56 8.89,35.56 | 8.89,35.56 8.89,43.18 KON-PROP1B.P$8 | 8.89,35.56 8.89,33.02 CF1.2 | CF2.2 41.91,33.02 41.91,35.56 | CF3.2 80.01,33.02 80.01,35.56
PODSVET-K-B1
  Bottom 0.813: KON-PROP1A.P$8 87.63,76.2 87.63,80.01 KON-DIS2K.P$1
PODSVET-K-B3  (via drill 0.7)
  Top 0.813: v18.41,5.08 18.41,15.24 KON-PROP2B.P$6
  Bottom 0.813: 62.23,10.16 62.23,27.94 | 62.23,27.94 73.66,27.94 KON-DIS1.16 | MOD4.LCD_LED_K 62.23,10.16 | 62.23,10.16 62.23,5.08 v18.41,5.08 | CF5.2 62.23,33.02 62.23,27.94
ROT-CLK
  Top 0.813: SW2.B 41.91,75.56 41.91,78.11 59.69,78.11 MOD1.D2
ROT-DT
  Top 0.813: MOD1.D3 57.15,82.55 34.8,82.55 SW2.A
ROT-TL  (via drill 0.7)
  Top 0.813: v52.07,76.2 44.45,76.2 44.45,73.03 20.32,73.03 SW2.SW+
  Bottom 0.813: v52.07,76.2 52.07,80.01 54.61,80.01 MOD1.D4
SEC-SELC
  Top 0.813: SW1.P20SMD SW1.P20 SW1.P10 SW1.P10SMD
  Bottom 0.813: MOD1.D6 49.53,93.98 SW1.P20
VLHKOMER
  Top 0.813: KON-PROP2A.P$4 77.47,53.34 77.47,38.1 11.43,38.1 11.43,46.99 7.62,46.99 7.62,50.8 KON-PROP1B.P$5
VLHKOMER-B1  (via drill 0.7)
  Top 0.813: v49.53,74.3 88.9,74.3 88.9,83.82 KON-PROP1A.P$5
  Bottom 0.813: MOD1.D5 52.07,82.55 49.53,82.55 v49.53,74.3
VLHKOMER-B3
  Top 0.813: AM2302.DATA 88.9,24.13 83.82,24.13 83.82,30.48 66.04,30.48 | 66.04,30.48 36.83,30.48 | 36.83,30.48 12.7,30.48 | 12.7,30.48 12.7,20.32 KON-PROP2B.P$4 | CF1.1 12.7,33.02 12.7,30.48 | CF2.1 36.83,33.02 36.83,30.48 | CF3.1 66.04,33.02 66.04,30.48
VO-VEE  (via drill 0.7)
  Top 0.813: KON-DIS1.3 v66.04,10.16 | v66.04,15.24 26.67,15.24 MOD4.LCD_VEE
  Bottom 0.813: v66.04,10.16 v66.04,15.24

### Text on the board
Top: Ver:1.2 | Mesicni hodiny / s meteostanici
tPlace: 1 | GND | SCL | V | T | P | SELC | SEC | SDA | VCC | VLH | GND | L-A | DATA | Arduino NANO | L-K | Vcc | 1 | 1 | EEPROM | SCL | GND | SDA | SCL | VCC | SDA | TLAK | EERAM | VLH | VCC | VLH | L-K | L-A | RTC | L-A | GND | GND | L-K | PWR | +5V | 1 | SCL | SDA | VCC | VLH | L-K | I2C-DISPLAY | L-A | GND | 1
bPlace: 1 | SELC | R | SEC | G | V | T | P | B | DS18B20 | Rotator | LED | 1 | 1 | 1 | LED | VLHKOST | 1 | TEPLOTA-IN | DISPLAY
